FUNCTION_BLOCK p03_IL_logOperacije
VAR_INPUT
END_VAR
VAR_OUTPUT
END_VAR
VAR
END_VAR

VAR_INPUT
	x1: BOOL;
	x2: BOOL;
END_VAR

VAR_OUTPUT
	yNot: BOOL;
	yAnd: BOOL;
	yOr: BOOL;
END_VAR

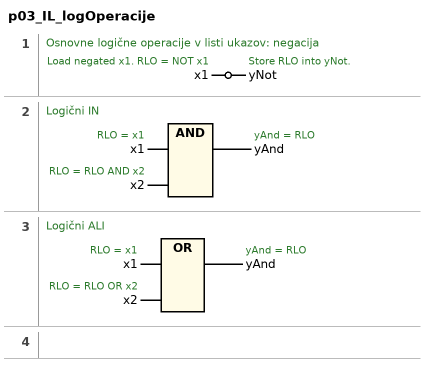
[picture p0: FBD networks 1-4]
// NETWORK 1
// Osnovne logične operacije v listi ukazov: negacija
//   x1: Load negated x1. RLO = NOT x1
//   yNot: Store RLO into yNot.
yNot := NOT x1;

// NETWORK 2
// Logični IN
//   x1: RLO = x1
//   x2: RLO = RLO AND x2
//   yAnd: yAnd = RLO
yAnd := x1 AND x2;

// NETWORK 3
// Logični ALI
//   x1: RLO = x1
//   x2: RLO = RLO OR x2
//   yAnd: yAnd = RLO
yAnd := x1 OR x2;

// NETWORK 4
// instruction list

END_FUNCTION_BLOCK
